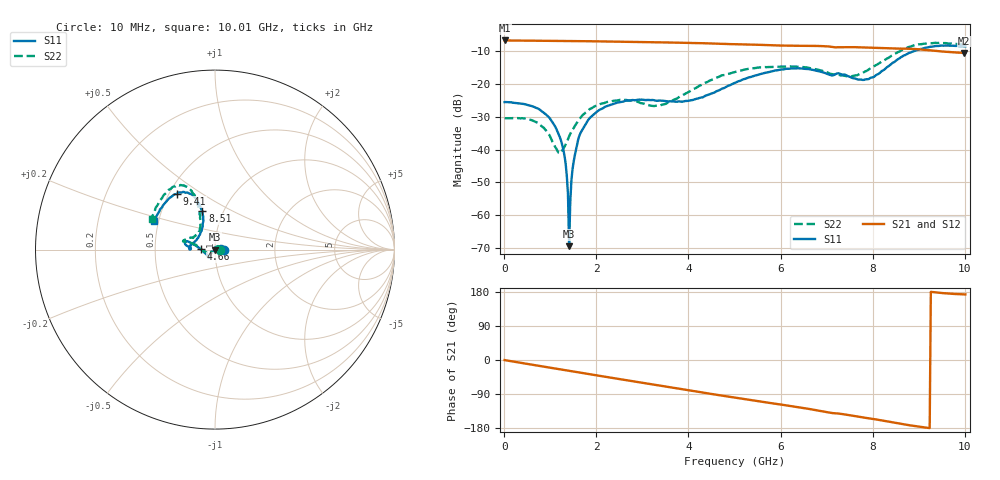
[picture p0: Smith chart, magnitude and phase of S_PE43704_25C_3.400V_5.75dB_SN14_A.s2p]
! Device ID: PE43704
! Dir: z:\PE43704\PE43704_Char_1_20130516\PE43704\AMB\3p400V\5p75dB
! Serial: 14
! Insertion: A
! Impedance: 50 ohm
! Temp: Amb
! VDD: 3.400V
! Attenuation Step: 5.75dB
! IDD: 1.140560e-01mA
#  Hz  S  RI  R  50
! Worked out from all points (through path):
!   401 points, 10 MHz to 10.01 GHz, reference 50 ohm
!   highest |S21| = -6.79 dB at 10 MHz (marker M1); lowest = -10.6 dB at 9.985 GHz (marker M2)
!   group delay of S21, straight-line fit = 53.3 ps
!   lowest |S11| = -69.4 dB at 1.41 GHz (marker M3), VSWR 1.00, Z = 50 + j0.0335 ohm
!   |S11| at or under -10 dB: start of sweep to 8.895 GHz
!   |S22| runs from -41.1 to -7.5 dB; largest |S21 - S12| = 0.0035
!   S11 on the Smith chart (normalised r, x): 10 MHz: 1.11, +0.00; 4.66 GHz: 0.85, +0.00; 8.51 GHz: 0.80, +0.36; 9.41 GHz: 0.55, +0.40; 10.01 GHz: 0.47, +0.17
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1e7  0.0527 0.000226  0.4578 -0.00189  0.4578 -0.00185  0.0299 0.000269
6.85e8  0.0383 0.0206  0.44 -0.1098  0.4399 -0.1096  0.0179 0.0194
1.035e9  0.0212 0.0165  0.4219 -0.1619  0.4218 -0.1617  0.00269 0.0136
1.26e9  0.00869 0.00797  0.4062 -0.1945  0.4063 -0.1943  -0.00858 0.00447
1.385e9  0.0011 0.00178  0.3964 -0.2114  0.3965 -0.2113  -0.0142 -0.00211
1.41e9  -4.66e-05 0.000335  0.3944 -0.2148  0.3944 -0.2147  -0.0155 -0.0036
1.46e9  -0.00257 -0.00225  0.3903 -0.2214  0.3903 -0.2212  -0.0174 -0.00648
1.485e9  -0.00388 -0.00328  0.3883 -0.2248  0.3883 -0.2247  -0.0186 -0.00777
1.535e9  -0.00621 -0.00545  0.384 -0.2312  0.384 -0.231  -0.0203 -0.0106
1.685e9  -0.0137 -0.0136  0.3702 -0.2507  0.3703 -0.2505  -0.026 -0.0192
2.235e9  -0.0293 -0.0354  0.3121 -0.3126  0.3123 -0.3125  -0.0359 -0.039
3.36e9  -0.0357 -0.0426  0.1662 -0.3951  0.1666 -0.3948  -0.0402 -0.0233
4.66e9  -0.0794 0.00175  -0.0194 -0.408  -0.019 -0.408  -0.1237 0.0331
5.01e9  -0.1019 0.0184  -0.0645 -0.3963  -0.0641 -0.3966  -0.1475 0.0353
6.685e9  -0.1624 0.0255  -0.2465 -0.2873  -0.2466 -0.287  -0.1616 0.0581
7.585e9  -0.113 0.0444  -0.3054 -0.1945  -0.3049 -0.1942  -0.09 0.0983
7.935e9  -0.082 0.089  -0.3221 -0.155  -0.3222 -0.1558  -0.082 0.1486
8.36e9  -0.0659 0.1779  -0.3326 -0.1019  -0.3322 -0.1035  -0.0916 0.2376
8.51e9  -0.0705 0.2158  -0.3348 -0.0811  -0.3342 -0.0836  -0.1025 0.2758
9.41e9  -0.213 0.3105  -0.3158 0.012  -0.3154 0.0126  -0.2477 0.3383
9.985e9  -0.3323 0.1687  -0.2937 0.0356  -0.2948 0.0367  -0.3481 0.1781
1.001e10  -0.3378 0.1583  -0.2946 0.0357  -0.2965 0.0361  -0.3521 0.1695
